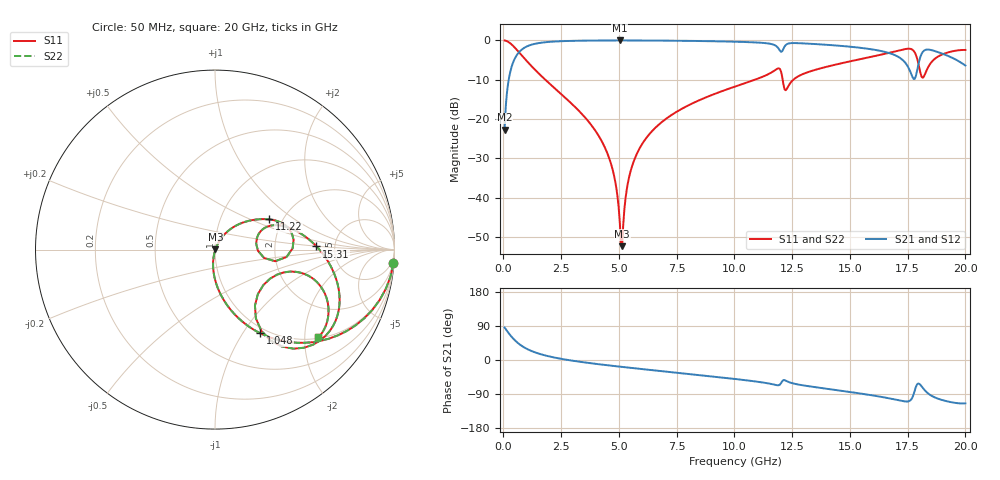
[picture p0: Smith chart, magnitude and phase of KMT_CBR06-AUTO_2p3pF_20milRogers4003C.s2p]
! Data measured by Modelithics Inc. support@modelithics.com 813-866-6335
! KEMET CBR06-AUTO 2.3pF, Pad Width= 0.851mm, Pad Length= 0.64mm, Pad Gap= 0.62mm, 20mil Rogers 4003C substrate Data, January 2022
# hz S ma R 50
! 2 Port Network Data from SP1.SP block
! freq  magS11  angS11  magS21  angS21  magS12  angS12  magS22  angS22
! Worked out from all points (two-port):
!   401 points, 50 MHz to 20 GHz, reference 50 ohm
!   highest |S21| = -0.02 dB at 5.037 GHz (marker M1); lowest = -22.7 dB at 50 MHz (marker M2)
!   |S21| within 3 dB of the highest: 673.1 MHz to 16.57 GHz (15.9 GHz wide, 184 % of centre); 18.15 GHz to 18.83 GHz (685.4 MHz wide, 3.71 % of centre)
!   lowest |S11| = -52.4 dB at 5.137 GHz (marker M3), VSWR 1.00, Z = 50.2 + j0.0574 ohm
!   |S11| at or under -10 dB: 1.809 GHz to 10.89 GHz (9.081 GHz wide, 143 % of centre); 12.09 GHz to 12.55 GHz (466.4 MHz wide, 3.79 % of centre)
!   |S22| runs from -52.4 to 0.0 dB; largest |S21 - S12| = 0
!   S11 on the Smith chart (normalised r, x): 50 MHz: 1, -26; 1.048 GHz: 0.93, -1.20; 11.22 GHz: 1.70, +0.65; 15.31 GHz: 3.60, +0.19; 20 GHz: 1.03, -2.34
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5e7  0.9973 -4.4  0.07299 85.6  0.07299 85.6  0.9973 -4.4
3.99125e8  0.8618 -31.8  0.5062 58.1  0.5062 58.1  0.8618 -31.8
1.0475e9  0.5307 -61.5  0.8463 28.3  0.8463 28.3  0.5307 -61.5
3.391625e9  0.116 -94.5  0.9914 -5.4  0.9914 -5.4  0.116 -94.5
4.588625e9  0.031 -100.9  0.9974 -14.5  0.9974 -14.5  0.031 -100.9
4.838e9  0.01607 -99.1  0.9977 -16.2  0.9977 -16.2  0.01607 -99.1
5.0375e9  0.004829 -82.8  0.9978 -17.6  0.9978 -17.6  0.004829 -82.8
5.13725e9  0.002403 13.7  0.9978 -18.3  0.9978 -18.3  0.002403 13.7
5.386625e9  0.01525 62.2  0.9976 -19.9  0.9976 -19.9  0.01525 62.2
5.636e9  0.02865 64.2  0.9973 -21.6  0.9973 -21.6  0.02865 64.2
6.73325e9  0.08508 59.8  0.9938 -28.6  0.9938 -28.6  0.08508 59.8
1.0025e10  0.2584 39.1  0.962 -50.1  0.962 -50.1  0.2584 39.1
1.1222e10  0.3445 29.3  0.9296 -59.3  0.9296 -59.3  0.3445 29.3
1.206988e10  0.3415 -10.9  0.7286 -56.0  0.7286 -56.0  0.3415 -10.9
1.226938e10  0.2416 15.3  0.895 -55.9  0.895 -55.9  0.2416 15.3
1.336662e10  0.4107 18.3  0.9027 -70.5  0.9027 -70.5  0.4107 18.3
1.531175e10  0.5657 1.8  0.8135 -87.1  0.8135 -87.1  0.5657 1.8
1.670825e10  0.6951 -13.7  0.6884 -101.2  0.6884 -101.2  0.6951 -13.7
1.775562e10  0.7388 -47.7  0.3237 -91.0  0.3237 -91.0  0.7388 -47.7
1.805488e10  0.3834 -54.5  0.6206 -65.8  0.6206 -65.8  0.3834 -54.5
1.845388e10  0.4918 -15.1  0.7608 -91.3  0.7608 -91.3  0.4918 -15.1
2e10  0.7554 -40.3  0.4784 -114.3  0.4784 -114.3  0.7554 -40.3
